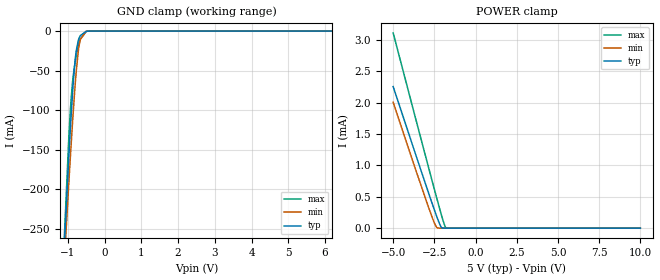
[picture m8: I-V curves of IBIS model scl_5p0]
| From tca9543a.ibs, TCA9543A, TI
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|   scl_5p0 Model
[Model]   scl_5p0
Model_type   Input
Vinl = 1.5
Vinh = 3.5
|   typ   min   max
|   (nom PVT)   (fast PVT)   (slow PVT)
C_comp   1.029e-11   7.571e-12   1.173e-11
[Model spec]
|subparameter
Vinl   1.5   1.35   1.65
Vinh   3.5   3.15   3.85
| Where nom  PVT is Nominal Process, 5V, 27C
|   Fast PVT is Strong Process,  5.5V, -40C
|   Slow PVT is Weak Process,   4.5V, 85C
[Voltage Range]   5   4.5   5.5
|Junction Temperature
[Temperature Range]   27   85   -40
[Power Clamp Reference]   5   4.5   5.5
[GND Clamp Reference]   0   0   0
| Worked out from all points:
|   GND clamp passes 1 mA (typ) near -0.52 V on its own axis
[GND Clamp]
|   Voltage   I(typ)   I(min)   I(max)
-5V       -4.363A    -3.897A    -4.959A
-1.125V   -299.5mA   -317.2mA   -292.1mA
-974mV    -160.7mA   -193.5mA   -136.7mA
-924.5mV  -119mA     -155mA     -95.94mA
-875mV    -81.2mA    -118.3mA   -66.27mA
-855.5mV  -67.85mA   -104.5mA   -57.8mA
-815mV    -44.03mA   -77.52mA   -43.91mA
-779mV    -28.26mA   -55.96mA   -33.89mA
-693.5mV  -9.061mA   -18.64mA   -15.24mA
-662mV    -5.874mA   -10.77mA   -10.29mA
-500mV    -352.7uA   -288.9uA   -483.3uA
10V       0A         0A         0A
[POWER Clamp]
|   Voltage   I(typ)   I(min)   I(max)
-5V       2.258mA    2.008mA    3.114mA
-3.042V   709.9uA    476.2uA    1.157mA
-2.494V   287.8uA    80.47uA    615.1uA
-2.327V   165.6uA    7.111uA    453.1uA
-2.09V    19.61uA    0A         227.7uA
-2.02V    2.926uA    0A         163.7uA
-1.876V   15.26nA    0A         44.66uA
-1.788V   0A         0A         4.124uA
10V       0A         0A         0A
